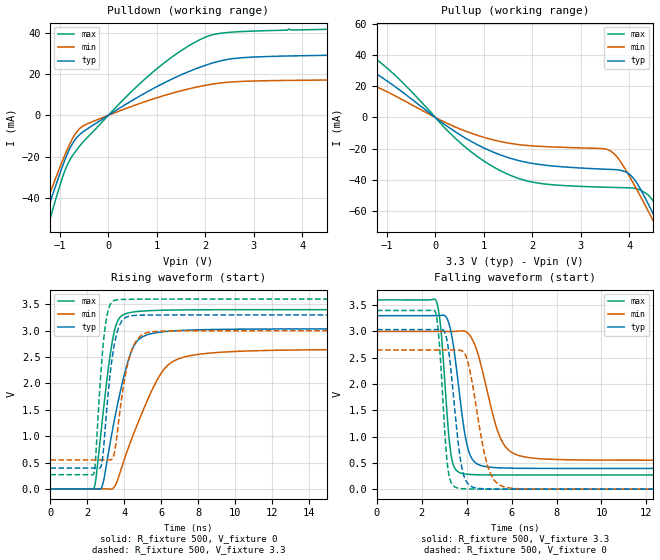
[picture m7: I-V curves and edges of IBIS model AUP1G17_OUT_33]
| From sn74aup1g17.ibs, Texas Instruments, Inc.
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[Model]   AUP1G17_OUT_33
Model_type  Output
Vref =   0
Rref =   1E6
Cref =   30p
Vmeas =   1.65
| variable   typ   min   max
C_comp   2.81pF   1.90pF   4.21pF
| C_pullup   3.21pF   1.90pF   4.21pF
| C_pulldown   2.42pF   2.21pF   2.99pF
[Temperature Range]   40   100   -40
| Ambient temperature   25   85   -40
[Voltage range]   3.3   3   3.6
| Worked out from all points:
|   slope of the pulldown table from 0 to 0.495 V, typ, clamps not added: 68.4 ohm
|   slope of the pullup table from 0 to 0.495 V, typ, clamps not added: 45.8 ohm
|   rising waveform, R_fixture 500, V_fixture 0: 20-80 % time 1.1ns typ, 1.89ns min, 694ps max; typ from 0 V to 3.04 V
|   falling waveform, R_fixture 500, V_fixture 3.3: 20-80 % time 537ps typ, 892ps min, 349ps max; typ from 3.3 V to 0.394 V
|   rising waveform, R_fixture 500, V_fixture 3.3: 20-80 % time 521ps typ, 677ps min, 407ps max; typ from 0.394 V to 3.3 V
|   falling waveform, R_fixture 500, V_fixture 0: 20-80 % time 449ps typ, 671ps min, 303ps max; typ from 3.04 V to 0 V
[Pulldown]
| AUP1G17_OUT_33
|   Voltage   I(typ)   I(min)   I(max)
-3.6V     -218.7mA   -196.3mA   -248.6mA
-1.515V   -64.37mA   -57.31mA   -75.82mA
-1.39V    -55.35mA   -49.29mA   -65.41mA
-1.275V   -47.14mA   -42mA      -55.89mA
-870mV    -19.93mA   -17.62mA   -25.18mA
-720mV    -12.85mA   -10.38mA   -18.82mA
-545mV    -8.444mA   -5.509mA   -13.51mA
940mV     13.13mA    8.018mA    21.36mA
1.5V      19.56mA    11.86mA    31.27mA
2.045V    24.53mA    14.67mA    38.2mA
3.1V      28.27mA    16.63mA    40.81mA
7.2V      29.73mA    17.36mA    42.67mA
[Pullup]
| AUP1G17_OUT_33
|   Voltage   I(typ)   I(min)   I(max)
-3.6V     42.88mA    27.27mA    57.92mA
-2.465V   31.53mA    19.52mA    45.85mA
-1.53V    32.87mA    22.09mA    44.95mA
-755mV    18.1mA     12.64mA    24.89mA
555mV     -11.98mA   -7.942mA   -17.3mA
1.65V     -27.07mA   -17.13mA   -38.31mA
3.61V     -33.32mA   -21.39mA   -44.82mA
4.08V     -38.63mA   -41.77mA   -45.28mA
4.375V    -54.25mA   -58.9mA    -49.24mA
4.565V    -66.24mA   -70.37mA   -57.33mA
4.775V    -80.02mA   -83.29mA   -71.37mA
7.2V      -250.7mA   -240.9mA   -257mA
[Ramp]
| AUP1G17_OUT_33
| variable   typ   min   max
dV/dt_r   1.82/1.10E-09   1.59/1.89E-09   2.04/6.96E-10
dV/dt_f   1.75/5.44E-10   1.48/8.96E-10   2.01/3.58E-10
R_load = 500
[Rising Waveform]
| AUP1G17_OUT_33
R_fixture =   500
C_fixture =   0
L_fixture =   0
V_fixture =   0
V_fixture_min = 0
V_fixture_max = 0
|   Time   V(typ)   V(min)   V(max)
0s        24.73nV    82.54nV    2.123nV
2.365ns   416.3uV    -27.44uV   15.86mV
2.82ns    69.96mV    697.3uV    1.328V
3.375ns   1.139V     6.166mV    2.841V
3.655ns   1.635V     185.1mV    3.194V
4.12ns    2.322V     679.6mV    3.327V
4.74ns    2.819V     1.252V     3.365V
5.955ns   2.974V     2.173V     3.387V
7.47ns    3.011V     2.52V      3.395V
30.7ns    3.035V     2.647V     3.399V
[Falling Waveform]
| AUP1G17_OUT_33
R_fixture =   500
C_fixture =   0
L_fixture =   0
V_fixture =   3.3
V_fixture_min = 3
V_fixture_max = 3.6
|   Time   V(typ)   V(min)   V(max)
0s        3.3V       3V         3.6V
2.63ns    3.299V     3V         3.589V
2.845ns   3.306V     3V         3.05V
3.29ns    3.009V     2.999V     681.5mV
3.77ns    1.482V     3.011V     301.5mV
4.03ns    807mV      2.974V     284mV
4.35ns    516.3mV    2.753V     275.8mV
5.48ns    405.1mV    989.8mV    269.9mV
6.505ns   396.7mV    619.8mV    269.4mV
30.7ns    394.1mV    550mV      269.3mV
[Rising Waveform]
| AUP1G17_OUT_33
R_fixture =   500
C_fixture =   0
L_fixture =   0
V_fixture =   3.3
V_fixture_min = 3
V_fixture_max = 3.6
|   Time   V(typ)   V(min)   V(max)
0s        394.1mV    550mV      269.3mV
2.355ns   394.4mV    550.1mV    288.4mV
2.45ns    394.5mV    550.1mV    575.1mV
2.74ns    421.3mV    550.4mV    2.221V
2.935ns   1.002V     550.3mV    2.984V
3.215ns   2.11V      549.3mV    3.475V
3.475ns   2.765V     702.4mV    3.575V
4.27ns    3.276V     2.485V     3.596V
5.28ns    3.296V     2.967V     3.599V
30.7ns    3.3V       3V         3.6V
[Falling Waveform]
| AUP1G17_OUT_33
R_fixture =   500
C_fixture =   0
L_fixture =   0
V_fixture =   0
V_fixture_min = 0
V_fixture_max = 0
|   Time   V(typ)   V(min)   V(max)
0s        3.035V     2.647V     3.399V
2.595ns   3.035V     2.647V     3.379V
2.775ns   3.037V     2.647V     2.791V
3.15ns    2.756V     2.648V     425.6mV
3.575ns   1.049V     2.648V     24.06mV
3.795ns   384.2mV    2.627V     9.827mV
4.065ns   97mV       2.389V     4.022mV
4.925ns   4.435mV    449.8mV    320.8uV
5.755ns   605.1uV    33.27mV    47.62uV
30.7ns    -27.86nV   32.96nV    -37.41nV
